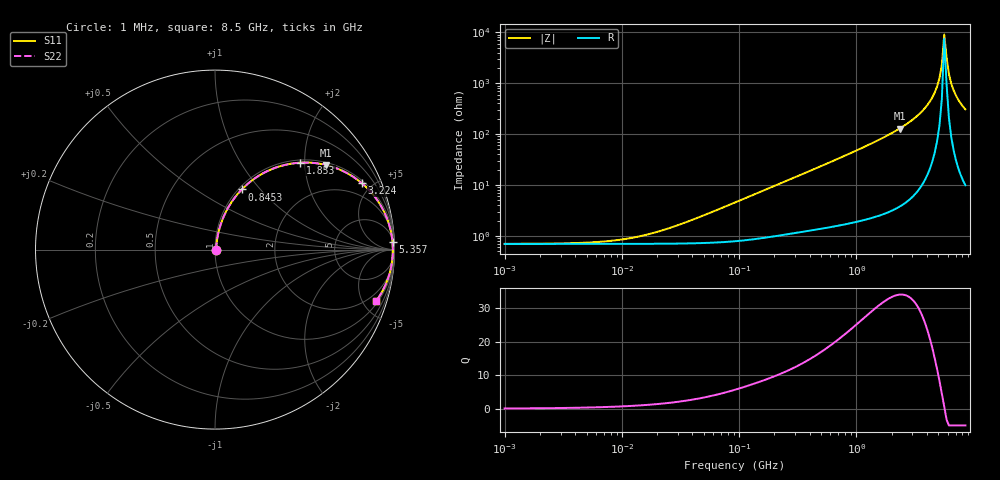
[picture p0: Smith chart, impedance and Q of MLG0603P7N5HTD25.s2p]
! S-Parameter Data Generated by TDK Corporation
! Copyright(C) 2025 TDK Corporation.
! All Rights Reserved.
! TDK P/N: MLG0603P7N5HTD25 (SMD / SMT Inductor (Coil))
! Property: L=7.5nH at 500MHz
! Size(LxWxT): 0.6x0.3x0.3mm
! Model Type: s2p (Touchstone File Format Version 1.0)
! Frequency: DC=Yes Start=1MHz Stop=8500MHz 198points Log-sweep
! Model Generated on Feb. 6, 2025
! Terms and conditions regarding TDK Simulation Models:
! 1)This simulation model is being provided solely for informational
!  purposes. Please refer to the specifications of the products in
!  terms of detailed characteristics of such products.
! 2)In no event shall TDK Corporation of any of its subsidiaries be
!  liable for any loss or damage arising, directly or indirectly,
!  from any information contained in this simulation model, including,
!  but not limited to loss or damages arising from any inaccuracies,
!  omissions or errors in connection with such information.
! 3)Any and all copyrights on this simulation model are owned by
!  TDK Corporation.  Duplication or redistribution of this simulation
!  model without prior written permission from TDK Corporation
!  is prohibited.
! 4)This simulation model is subject to any modification or change
!  without any prior notice.
! 5)Neither TDK Corporation nor any of its subsidiaries shall make any
!  warranty, express or implied, including but not limited to the
!  correctness, implied warranties of merchantability and fitness for
!  a particular purpose with respect to this simulation models.
! 6)The use of this simulation model shall be deemed to have consented
!  to the terms and conditions hereof.
! Port Assignments:
!  1 ---@@@--- 2
! Applicable Conditions:
!  Temperature = 25 degC
!  DC Bias Current = 0 A
!  Small Signal Operation
# Hz S MA R 50
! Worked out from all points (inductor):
!   197 points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, 1 MHz to 8.5 GHz, reference 50 ohm
!   read as one part in series: L = 7.77 nH near 46.13 MHz
!   highest Q = 34.1 at 2.334 GHz (marker M1), where L = 8.78 nH
!   self-resonance near 5.61 GHz
!   S11 on the Smith chart (normalised r, x): 1 MHz: 1.01, +0.00; 845.3 MHz: 1.03, +0.80; 1.853 GHz: 1.06, +1.90; 3.224 GHz: 1.14, +4.36; 5.357 GHz: 11, +45; 8.5 GHz: 1.20, -6.14
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1000000  0.006968 4.0  0.993 -0.0  0.993 -0.0  0.006968 4.0
4587603  0.007303 17.7  0.993 -0.1  0.993 -0.1  0.007303 17.7
1.053054e7  0.008646 36.0  0.993 -0.3  0.993 -0.3  0.008646 36.0
2.10461e7  0.0124 55.0  0.9929 -0.6  0.9929 -0.6  0.0124 55.0
9.219544e7  0.04513 77.5  0.9912 -2.5  0.9912 -2.5  0.04513 77.5
4.229561e8  0.1937 75.1  0.9685 -11.1  0.9685 -11.1  0.1937 75.1
8.453103e8  0.3666 66.0  0.9146 -21.5  0.9146 -21.5  0.3666 66.0
1.852819e9  0.6793 45.5  0.7134 -42.8  0.7134 -42.8  0.6793 45.5
1.940355e9  0.6996 43.9  0.6937 -44.4  0.6937 -44.4  0.6996 43.9
2.333852e9  0.7788 37.2  0.6048 -51.1  0.6048 -51.1  0.7788 37.2
3.224109e9  0.8982 24.3  0.4118 -63.9  0.4118 -63.9  0.8982 24.3
3.877948e9  0.9477 16.5  0.2839 -71.3  0.2839 -71.3  0.9477 16.5
4.453958e9  0.9732 10.5  0.1822 -76.3  0.1822 -76.3  0.9732 10.5
4.884749e9  0.9841 6.4  0.1126 -78.7  0.1126 -78.7  0.9841 6.4
5.115526e9  0.9876 4.4  0.07752 -78.6  0.07752 -78.6  0.9876 4.4
5.357206e9  0.9899 2.4  0.04257 -75.1  0.04257 -75.1  0.9899 2.4
5.610304e9  0.9909 0.3  0.01094 -33.4  0.01094 -33.4  0.9909 0.3
5.87536e9  0.9906 -1.7  0.03079 71.3  0.03079 71.3  0.9906 -1.7
6.152938e9  0.9889 -3.7  0.06553 78.4  0.06553 78.4  0.9889 -3.7
6.44363e9  0.986 -5.8  0.1007 79.1  0.1007 79.1  0.986 -5.8
7.066863e9  0.9762 -9.8  0.1707 77.1  0.1707 77.1  0.9762 -9.8
8.5e9  0.9419 -17.9  0.3069 70.3  0.3069 70.3  0.9419 -17.9
